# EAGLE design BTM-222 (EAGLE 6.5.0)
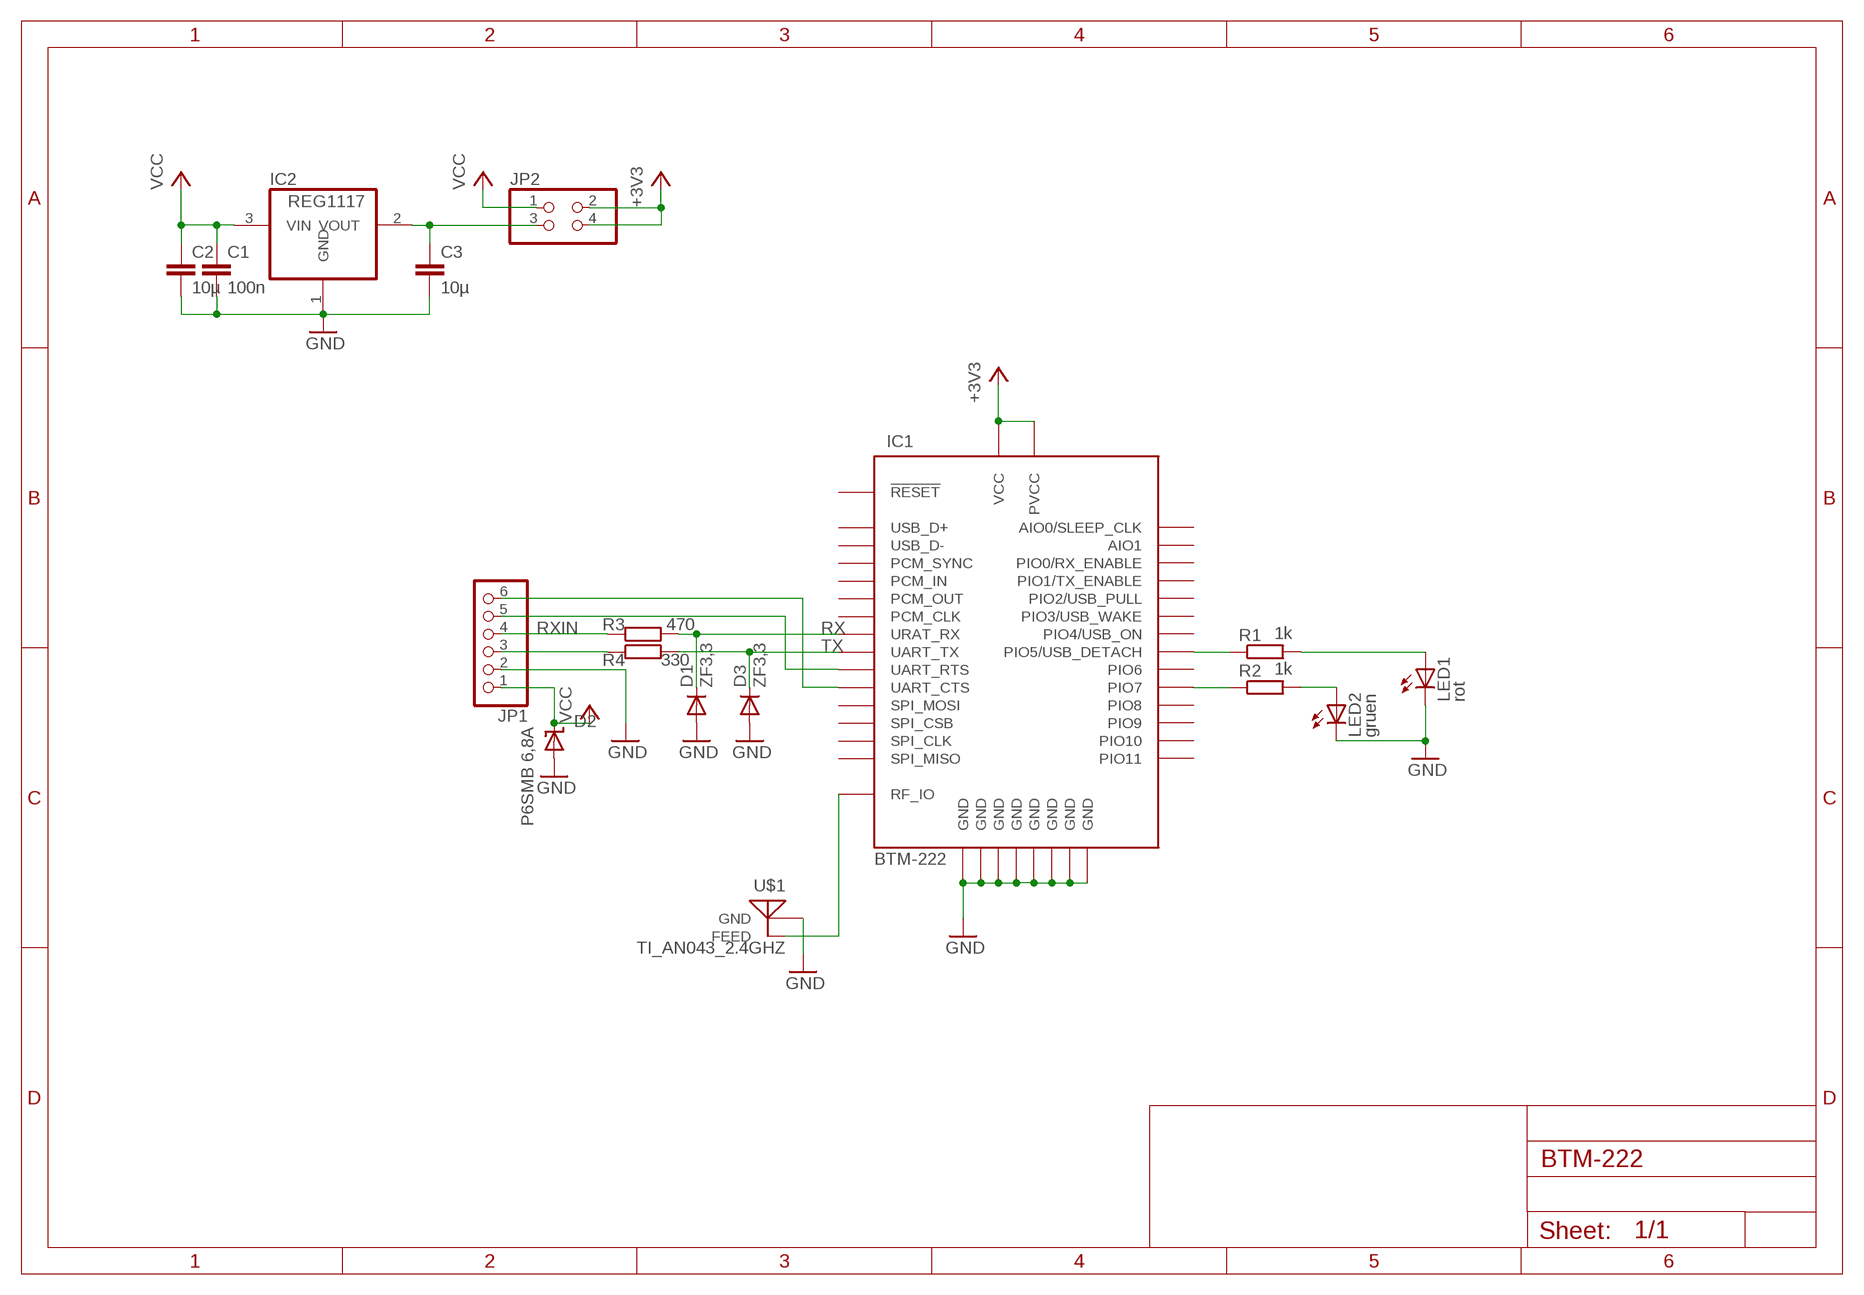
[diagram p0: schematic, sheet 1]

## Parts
C1  100n  C-EUC0805  [C0805]
C2  10µ  C-EUC0805  [C0805]
C3  10µ  C-EUC0805  [C0805]
D1  ZF3,3  DIODE-MINIMELF  [MINIMELF]
D2  P6SMB 6,8A  SUPPRESSOR-SMBJ  [SMBJ]
D3  ZF3,3  DIODE-MINIMELF  [MINIMELF]
IC1  BTM-222  [BTM-222]
IC2  REG1117  [SOT223]
JP1  PINHD-1X6  [1X06]
JP2  PINHD-2X2  [2X02]
LED1  rot  LG_T679-E1F1-1  [PLCC2]
LED2  gruen  LG_T679-E1F1-1  [PLCC2]
R1  1k  R-EU_R0805  [R0805]
R2  1k  R-EU_R0805  [R0805]
R3  470  R-EU_R0805  [R0805]
R4  330  R-EU_R0805  [R0805]
U$1  TI_AN043_2.4GHZ  [TI_AN043_2.4GHZ]

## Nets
+3V3: IC1.P$2(PVCC) IC1.P$17(VCC) JP2.2 JP2.4
GND: C1.2 C2.2 C3.2 D1.A D2.A D3.A IC1.P$1(GND) IC1.P$10(GND) IC1.P$18(GND) IC1.P$19(GND) IC1.P$29(GND) IC1.P$38(GND) IC1.P$39(GND) IC1.P$40(GND) IC2.1(GND) JP1.2 LED1.C LED2.C U$1.P$1(GND)
N$1: IC1.P$37(RF_IO) U$1.P$2(FEED)
N$2: LED1.A R1.2
N$3: LED2.A R2.2
N$4: IC1.P$28(UART_RTS) JP1.5
N$5: IC1.P$30(UART_CTS) JP1.6
N$6: JP1.3 R4.1
N$8: IC1.P$13(PIO7) R2.1
N$9: IC1.P$11(PIO5/USB_DETACH) R1.1
N$14: C3.1 IC2.2(VOUT) JP2.3
RX: D1.C IC1.P$26(URAT_RX) R3.2
RXIN: JP1.4 R3.1
TX: D3.C IC1.P$27(UART_TX) R4.2
VCC: C1.1 C2.1 D2.C IC2.3(VIN) JP1.1 JP2.1
Unconnected: IC1.P$3(AIO0/SLEEP_CLK) IC1.P$4(AIO1) IC1.P$5(PIO0/RX_ENABLE) IC1.P$6(PIO1/TX_ENABLE) IC1.P$7(PIO2/USB_PULL) IC1.P$8(PIO3/USB_WAKE) IC1.P$9(PIO4/USB_ON) IC1.P$12(PIO6) IC1.P$14(PIO8) IC1.P$15(PIO9) IC1.P$16(!RESET!) IC1.P$20(USB_D+) IC1.P$21(USB_D-) IC1.P$22(PCM_SYNC) IC1.P$23(PCM_IN) IC1.P$24(PCM_OUT) IC1.P$25(PCM_CLK) IC1.P$31(SPI_MOSI) IC1.P$32(SPI_CSB) IC1.P$33(SPI_CLK) IC1.P$34(SPI_MISO) IC1.P$35(PIO11) IC1.P$36(PIO10)

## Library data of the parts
C1-C3 = rcl:C-EU: CAPACITOR, European symbol
D1 D3 = diode:DIODE-: DIODE
D2 = diode:SUPPRESSOR-: Suppressor diode
IC1 = Bluetooth:BTM-222
IC2 = burr-brown:REG1117: 800mA and 1A Low Dropout (LDO) Positive Regulator 1.8V, 2.5V, 2.85V, 3.3V, 5V, and Adj; MPN: REG1117; OC_FARNELL: 1097566; OC_NEWARK: 14P6981
JP1 = pinhead:PINHD-1X6: PIN HEADER
JP2 = pinhead:PINHD-2X2: PIN HEADER
LED1 LED2 = led:*_T679-?-1: LC TOPLED® Low Current LED; COLOR: green
R1-R4 = rcl:R-EU_: RESISTOR, European symbol
U$1 = Bluetooth:TI_AN043_2.4GHZ

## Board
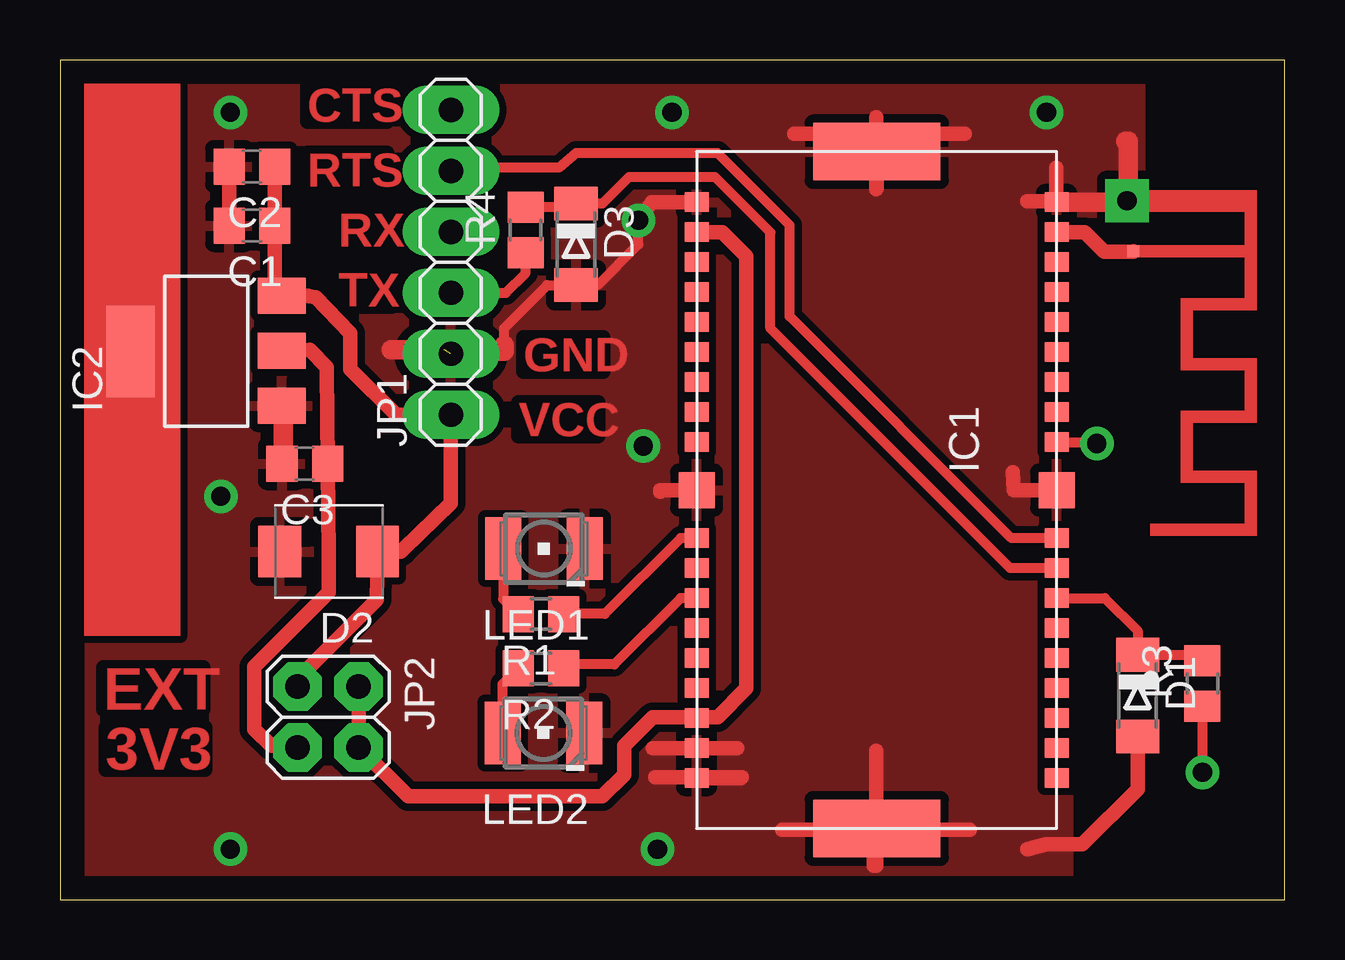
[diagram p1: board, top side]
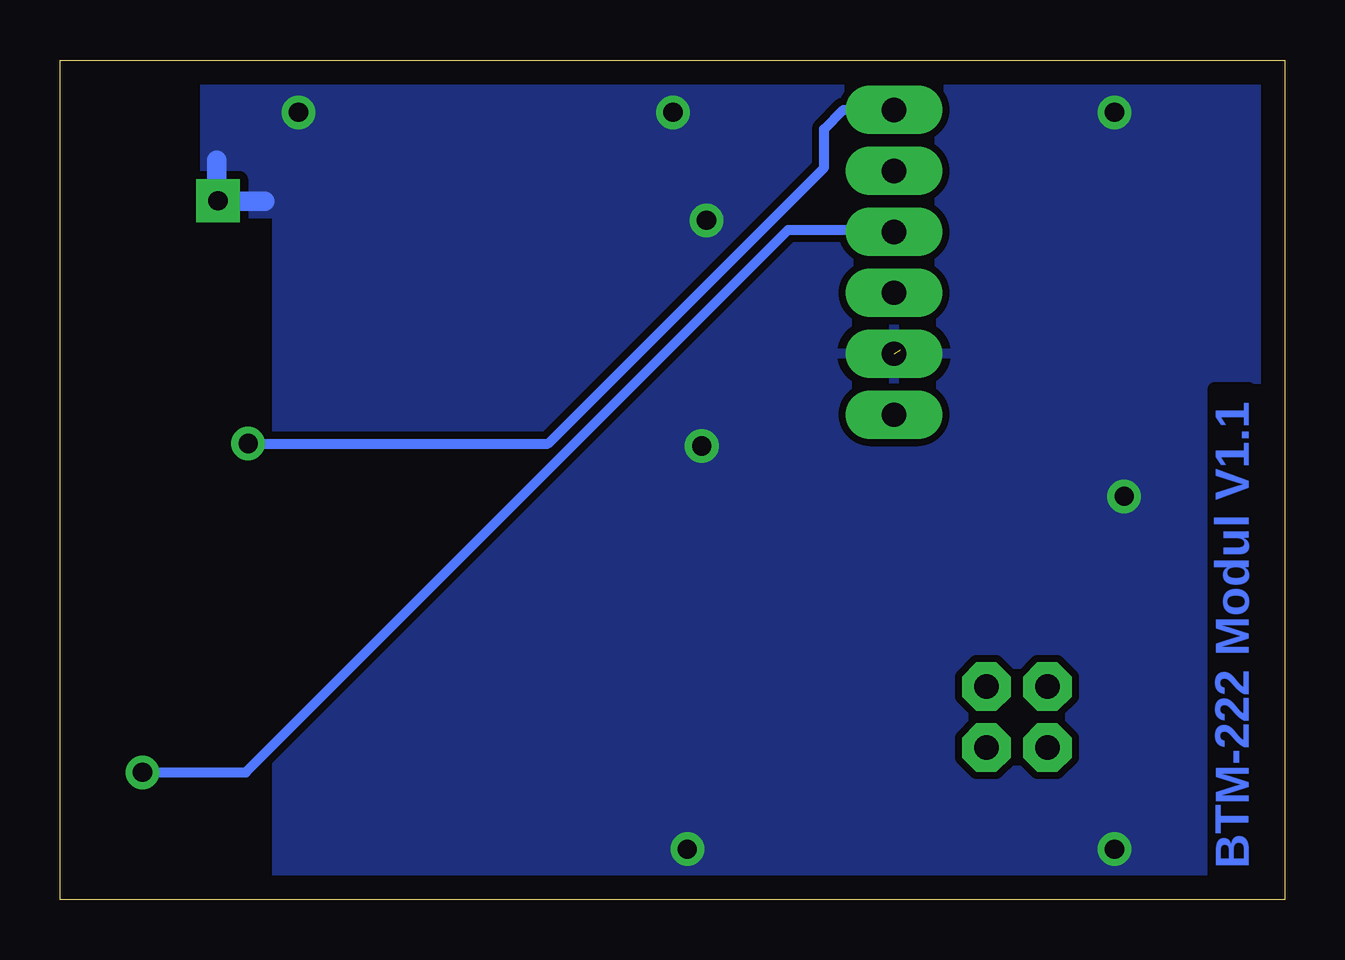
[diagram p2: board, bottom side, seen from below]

Size 51.04 x 34.98 mm. Coordinates in mm from the lower left corner, seen from the top.
Outline: 0,0 51.04,0 51.04,34.98 0,34.98 0,0
Copper layers (1*16): Top 0.035mm / dielectric 1.5mm / Bottom 0.035mm
Design rules "default": minimum track width 0.3mm, minimum drill 0.8mm, track to track 0.2mm, track to pad 0.2mm, pad to pad 0.2mm, via to via 0.2mm, smd to smd 0.2mm, copper to edge 1mm, drill to drill 1mm, minimum pad ring 0.5mm, minimum via ring 0.3mm, stop-mask expansion 4mil, vias tented up to drill 0mil, thermal gap 14mil

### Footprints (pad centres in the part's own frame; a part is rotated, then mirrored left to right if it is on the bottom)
C0805 = smd 1.3 x 1.5: 1 -0.95,0; 2 0.95,0
MINIMELF = smd 1.4 x 1.8: A 1.7,0; C -1.7,0
SMBJ = smd 1.78 x 2.16: A 2.04,0; C -2.03,0
BTM-222 = smd 0.8 x 1: P$1 -12,-7.5; P$2 -10.75,-7.5; P$3 -9.5,-7.5; P$4 -8.25,-7.5; P$5 -7,-7.5; P$6 -5.75,-7.5; P$7 -4.5,-7.5; P$8 -3.25,-7.5; P$9 -2,-7.5; P$11 2,-7.5; P$12 3.25,-7.5; P$13 4.5,-7.5; P$14 5.75,-7.5; P$15 7,-7.5; P$16 8.25,-7.5; P$17 9.5,-7.5; P$18 10.75,-7.5; P$19 12,-7.5; P$20 12,7.5; P$21 10.75,7.5; P$22 9.5,7.5; P$23 8.25,7.5; P$24 7,7.5; P$25 5.75,7.5; P$26 4.5,7.5; P$27 3.25,7.5; P$28 2,7.5; P$30 -2,7.5; P$31 -3.25,7.5; P$32 -4.5,7.5; P$33 -5.75,7.5; P$34 -7,7.5; P$35 -8.25,7.5; P$36 -9.5,7.5; P$37 -10.75,7.5; P$38 -12,7.5 | smd 1.5 x 1.5: P$10 0,-7.5; P$29 0,7.5 | smd 2.4 x 5.3: P$39 -14.1,0; P$40 14.1,0
SOT223 = smd 1.499 x 2.007: 1 -2.261,-3.15; 2 0.025,-3.15; 3 2.311,-3.15 | smd 3.81 x 2.007: 4 0,3.15
1X06 = drill 1.016 long: 1 -6.35,0; 2 -3.81,0; 3 -1.27,0; 4 1.27,0; 5 3.81,0; 6 6.35,0
2X02 = drill 1.016 octagon: 1 -1.27,-1.27; 2 -1.27,1.27; 3 1.27,-1.27; 4 1.27,1.27
PLCC2 = smd 2.6 x 1.5: A 0,1.7; C 0,-1.7
R0805 = smd 1.3 x 1.5: 1 -0.95,0; 2 0.95,0
TI_AN043_2.4GHZ = drill 0.8 pad 1.4 square: P$1 0.45,0 | smd 0.5 x 0.5: P$2 2.55,0.25

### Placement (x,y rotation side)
C1  8,28.08 180 top
C2  8,30.54 180 top
C3  10.2,18.16 180 top
D1  44.9,8.5 270 top
D2  11.2,14.5 180 top
D3  21.5,27.3 270 top
IC1  34.03,17.06 270 top
IC2  6.09,22.84 90 top
JP1  16.29,26.55 90 top
JP2  11.17,7.6 270 top
LED1  20.16,14.62 90 top
LED2  20.14,6.94 90 top
R1  20.04,11.89 180 top
R2  20.04,9.63 180 top
R3  47.6,9 90 top
R4  19.4,27.9 90 top
U$1  44.46,29.56 270 top

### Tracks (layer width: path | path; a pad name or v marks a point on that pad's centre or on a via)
+3V3
  Top 0.61: JP2.2 JP2.4 12.47,6.33 14.5,4.3 22.6,4.3 23.5,5.2 23.5,6.4 24.7,7.6 26.49,7.6 IC1.P$17 26.57,7.6 27.4,7.6 28.6,8.8 28.6,26.8 27.59,27.81 IC1.P$2
GND  (via drill 0.8)  (1 unrouted)
  Top 0.406: 44.46,29.06 U$1.P$1 | v24.1,28.3 24.1,27.3 22.4,25.6 D3.A 20.3,25.6 18.5,23.8 18.5,23.1
  Top 0.61: C2.2 C1.2 | IC2.1 9.27,20.55 C3.2 9.3,20.55 | IC1.P$29 39.74,17.06 39.7,17.8 | IC1.P$19 28.36,5.06 28.4,5.1 24.8,5.1 | IC1.P$18 28.21,6.31 28.2,6.3 24.7,6.3 | IC1.P$39 34.03,29.63 34,29.6 34,31.9 | 34,32.6 34,31.9 | 34,31.9 37.7,31.9 | 34,31.9 30.6,31.9 | IC1.P$40 34,3.66 | 34,3.66 34,6.2 | 34,3.66 34,1.4 33.9,1.4 33.9,2.9 | 33.9,2.9 37.9,2.9 | 33.9,2.9 30.1,2.9 | IC1.P$10 25,17.06 25,17 | IC1.P$1 24.66,29.06 v24.1,28.3 | D1.A 44.9,4.6 42.6,2.3 41.1,2.3 40.3,2.1 | 40.3,29.1 41.5,29.1 41.5,30.5
  Top 0.813: IC1.P$38 44.46,29.06 | 44.5,28.9 44.5,31.6 44.4,31.6 | 9.3,20.55 9.3,18.1 | JP1.2 18.5,22.84 18.5,23.1 | 16,22.9 13.8,22.9
  Bottom 0.61: v24.1,28.3 24,28.7 23.7,28.4
  Bottom 0.813: 42.5,29.1 44.5,29.1 44.5,30.8
  other vias: 7.1,32.8 6.7,16.8 7.1,2.1 24.9,2.1 24.3,18.9 41.1,32.8 25.5,32.8
  pour Top (isolate 0.305): 0,0 0,35 45,35 45,28.6 42,28.6 42,0
  pour Bottom (isolate 0.305): 0,0 0,35 45,35 45,28.6 42,28.6 42,0
N$1
  Top 0.61: IC1.P$37 42.69,27.81 43.5,27 U$1.P$2
N$2
  Top 0.406: LED1.A 18.46,12.52 R1.2
N$3
  Top 0.406: LED2.A 18.44,8.98 R2.2
N$4
  Top 0.406: IC1.P$28 39.64,15.06 30.4,24.3 30.4,28.1 27.4,31.1 21.5,31.1 20.8,30.5 16.03,30.5 JP1.5
N$5  (via drill 0.8)
  Top 0.406: IC1.P$30 43.2,19.06 v43.2,19
  Bottom 0.406: v43.2,19 30.7,19 19.2,30.5 19.2,32.1 18.4,32.9 JP1.6
N$6
  Top 0.406: JP1.3 18.58,25.28 19.4,26.1 R4.1
N$8
  Top 0.406: IC1.P$13 25.86,12.56 23.1,9.8 21.06,9.8 R2.1
N$9
  Top 0.406: IC1.P$11 25.86,15.06 22.7,11.9 R1.1
N$14
  Top 0.61: IC2.2 10.4,22.9 11.12,22.18 11.12,22.07 C3.1 11.15,17.95 11.2,14.4 11.2,12.8 8.1,9.7 8.1,7.1 8.8,6.4 9.83,6.4 JP2.3
RX
  Top 0.406: R3.2 47.35,10.2 D1.C 44.9,11.2 43.54,12.56 IC1.P$26
RXIN  (via drill 0.8)
  Top 0.406: R3.1 v47.6,5.3
  Bottom 0.406: v47.6,5.3 43.3,5.3 20.7,27.9 16.01,27.9 JP1.4
TX
  Top 0.406: IC1.P$27 39.59,13.81 29.6,23.8 29.6,27.8 27.3,30.1 23.7,30.1 22.6,29 D3.C 21.35,28.85 R4.2
VCC
  Top 0.61: C2.1 C1.1 8.95,25.44 IC2.3 10.2,25.15 | 10.2,25.15 10.35,25.15 | 10.2,25.15 10.65,25.1 12.1,23.6 12.1,22.1 14,20.2 JP1.1 16.29,16.52 14.3,14.6 14.2,14.5 D2.C 13.2,12.5 10.13,9.43 9.9,9.23 JP2.1
  Bottom 0.61: 16,20.29 JP1.1
(copper drawn outside any net)
  shapes: Top area x1

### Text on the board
Top: CTS | RTS | RX | TX | GND | VCC | EXT | 3V3
Bottom: BTM-222 Modul V1.1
